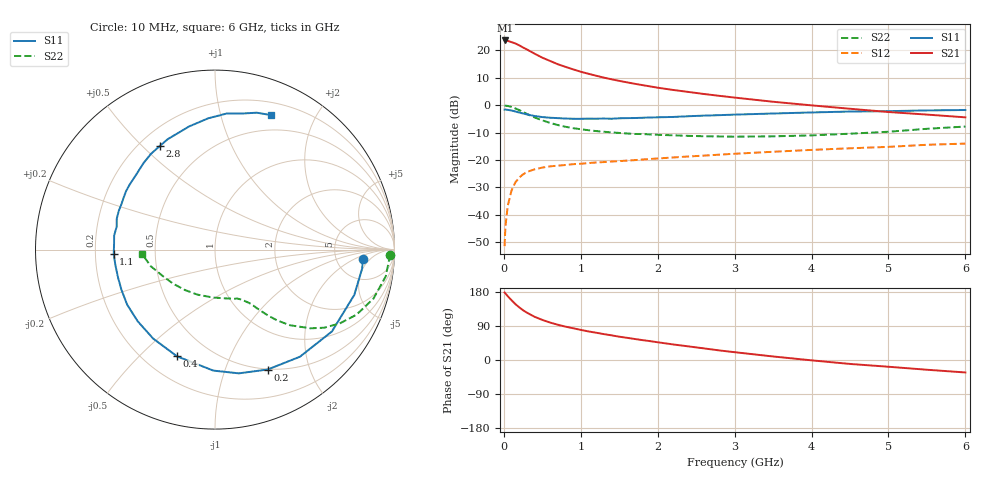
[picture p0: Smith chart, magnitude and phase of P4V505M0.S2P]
! SIEMENS Small Signal Semiconductors
! BFP182
! Si NPN RF Bipolar Junction Transistor in SOT143
! VCE = 0.5 V  IC = 5 mA
! Common Emitter S-Parameters:  March  1996
# GHz  S  MA  R  50
!  f  S11  S21  S12  S22
! GHz  MAG  ANG  MAG  ANG  MAG  ANG  MAG  ANG
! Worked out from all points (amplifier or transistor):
!   36 points, 10 MHz to 6 GHz, reference 50 ohm
!   highest |S21| = 23.5 dB at 20 MHz (marker M1)
!   |S21| within 3 dB of that: start of sweep to 280.8 MHz
!   unconditionally stable (mu >= 1): 1.271 GHz to end of sweep
!   at 250 MHz: K = 0.25, MSG = 23.1 dB, |S12| = -25.2 dB
!   at 1.4 GHz: K = 1.08, MAG = 13.2 dB, |S12| = -20.6 dB
!   at 6 GHz: K = 1.20, MAG = 2.1 dB, |S12| = -14.0 dB
!   S11 on the Smith chart (normalised r, x): 10 MHz: 9.46, -3.09; 200 MHz: 0.49, -1.41; 400 MHz: 0.33, -0.65; 1.1 GHz: 0.28, -0.02; 2.8 GHz: 0.28, +0.56; 6 GHz: 0.33, +1.45
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0.01  0.8258 -3.6  14.75 178.1  0.0027 88.3  0.9769 -1.7
0.02  0.8264 -7.4  14.96 176.0  0.006 87.2  0.9712 -3.6
0.05  0.8162 -18.0  14.72 168.5  0.0144 81.9  0.963 -8.9
0.1  0.7953 -35.0  13.96 157.8  0.0279 71.1  0.9241 -17.2
0.15  0.7616 -51.6  13.2 147.6  0.0391 62.4  0.8678 -24.7
0.2  0.7297 -66.3  12.21 138.9  0.0479 56.8  0.8078 -30.6
0.25  0.7021 -79.1  11.14 131.3  0.0548 51.1  0.7476 -35.6
0.3  0.6742 -90.8  10.27 124.9  0.0605 46.9  0.6895 -39.5
0.4  0.6311 -109.6  8.592 114.0  0.0675 40.0  0.5943 -45.2
0.5  0.6037 -124.8  7.28 105.8  0.0727 35.4  0.5256 -48.7
0.6  0.5873 -137.2  6.35 98.9  0.0765 32.7  0.4737 -51.1
0.7  0.5776 -147.9  5.537 93.1  0.0787 30.8  0.4327 -52.9
0.9  0.5622 -163.9  4.46 83.8  0.0838 28.3  0.3794 -55.5
1.1  0.5647 -177.6  3.705 75.4  0.0879 27.0  0.3482 -57.9
1.5  0.5737 162.6  2.753 61.5  0.0954 26.1  0.3103 -63.1
1.8  0.5862 150.1  2.306 52.5  0.1019 26.0  0.2961 -67.8
2.2  0.6067 136.1  1.881 41.1  0.111 25.2  0.2808 -75.9
2.8  0.654 118.1  1.471 25.3  0.125 23.0  0.268 -90.4
3.5  0.7008 102.0  1.147 9.3  0.1411 19.6  0.2692 -111.2
4.5  0.7613 85.0  0.855 -10.4  0.1632 13.7  0.3008 -140.9
5.5  0.7976 73.0  0.67 -25.7  0.189 7.7  0.3692 -165.4
6  0.8117 67.4  0.597 -32.9  0.1988 3.5  0.4059 -176.3
